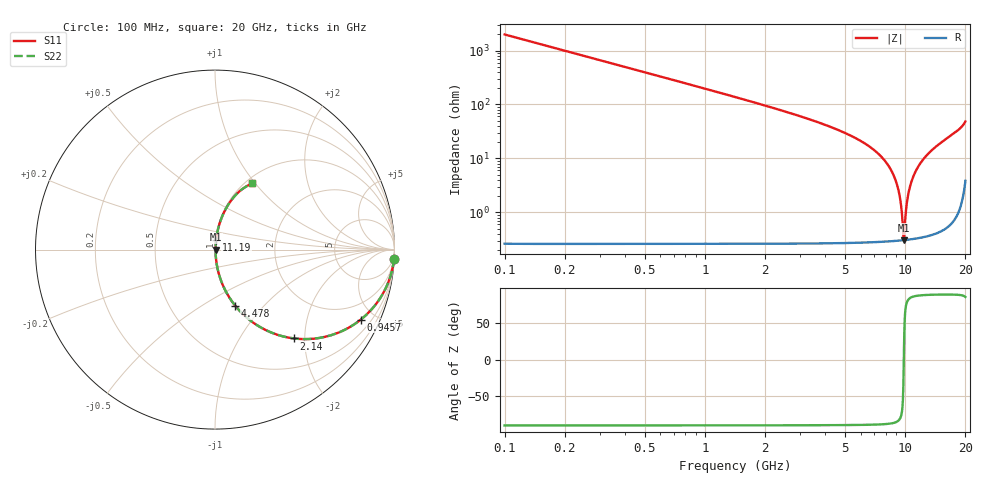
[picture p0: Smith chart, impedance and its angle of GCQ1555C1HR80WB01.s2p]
!Murata Part Number: GCQ1555C1HR80WB01
!These Parameters are Measured in Series Mode Connection
!Data Generated on Jan 08, 2026
!  o--ll--o
!Port1  Port2
!  o------o
!Operation Temp=25[degC], DC Bias Voltage=0[V]
!Freq. Start=100[MHz] Stop=20[GHz] 401[Steps]
# Hz S RI R 50
!Freq.(Hz) S11(Real) S11(Imag) S21(Real) S21(Imag) S12(Real) S12(Imag) S22(Real) S22(Imag)
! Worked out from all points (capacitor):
!   401 points, 100 MHz to 20 GHz, reference 50 ohm
!   read as one part in series: C = 800 fF near 199.5 MHz
!   lowest |Z| = 305 mohm at 9.851 GHz (marker M1)
!   series resonance near 9.852 GHz, so ESL is about 330 pH
!   S11 on the Smith chart (normalised r, x): 100 MHz: 1, -40; 945.8 MHz: 1.01, -4.17; 2.14 GHz: 1.01, -1.77; 4.478 GHz: 1.01, -0.71; 11.19 GHz: 1.01, +0.11; 20 GHz: 1.08, +0.97
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1e8  0.9975 -0.0501  0.00253 0.0501  0.00253 0.0501  0.9975 -0.0501
2.99e8  0.9778 -0.1471  0.0222 0.1471  0.0222 0.1471  0.9778 -0.1471
4.4825e8  0.9514 -0.2148  0.0486 0.2148  0.0486 0.2148  0.9514 -0.2148
9.4575e8  0.8126 -0.3896  0.1874 0.3896  0.1874 0.3896  0.8126 -0.3896
2.13975e9  0.4405 -0.495  0.5595 0.495  0.5595 0.495  0.4405 -0.495
3.43325e9  0.2081 -0.4034  0.7919 0.4034  0.7919 0.4034  0.2081 -0.4034
4.478e9  0.1135 -0.3134  0.8865 0.3134  0.8865 0.3134  0.1135 -0.3134
6.7665e9  0.0268 -0.1528  0.9732 0.1528  0.9732 0.1528  0.0268 -0.1528
8.10975e9  0.00928 -0.0797  0.9907 0.0797  0.9907 0.0797  0.00928 -0.0797
8.9555e9  0.00449 -0.0393  0.9955 0.0393  0.9955 0.0393  0.00449 -0.0393
9.453e9  0.00328 -0.0171  0.9967 0.0171  0.9967 0.0171  0.00328 -0.0171
9.60225e9  0.00312 -0.0106  0.9969 0.0106  0.9969 0.0106  0.00312 -0.0106
9.80125e9  0.00304 -0.00214  0.997 0.00214  0.997 0.00214  0.00304 -0.00214
9.851e9  0.00304 -4.51e-05  0.997 4.51e-05  0.997 4.51e-05  0.00304 -4.51e-05
9.9505e9  0.00307 0.00412  0.9969 -0.00412  0.9969 -0.00412  0.00307 0.00412
1.005e10  0.00313 0.00825  0.9969 -0.00825  0.9969 -0.00825  0.00313 0.00825
1.019925e10  0.00329 0.0144  0.9967 -0.0144  0.9967 -0.0144  0.00329 0.0144
1.0448e10  0.00371 0.0244  0.9963 -0.0244  0.9963 -0.0244  0.00371 0.0244
1.119425e10  0.0061 0.0534  0.9939 -0.0534  0.9939 -0.0534  0.0061 0.0534
1.338325e10  0.0213 0.131  0.9787 -0.131  0.9787 -0.131  0.0213 0.131
1.67165e10  0.0666 0.2384  0.9334 -0.2384  0.9334 -0.2384  0.0666 0.2384
2e10  0.2084 0.3684  0.7916 -0.3684  0.7916 -0.3684  0.2084 0.3684
